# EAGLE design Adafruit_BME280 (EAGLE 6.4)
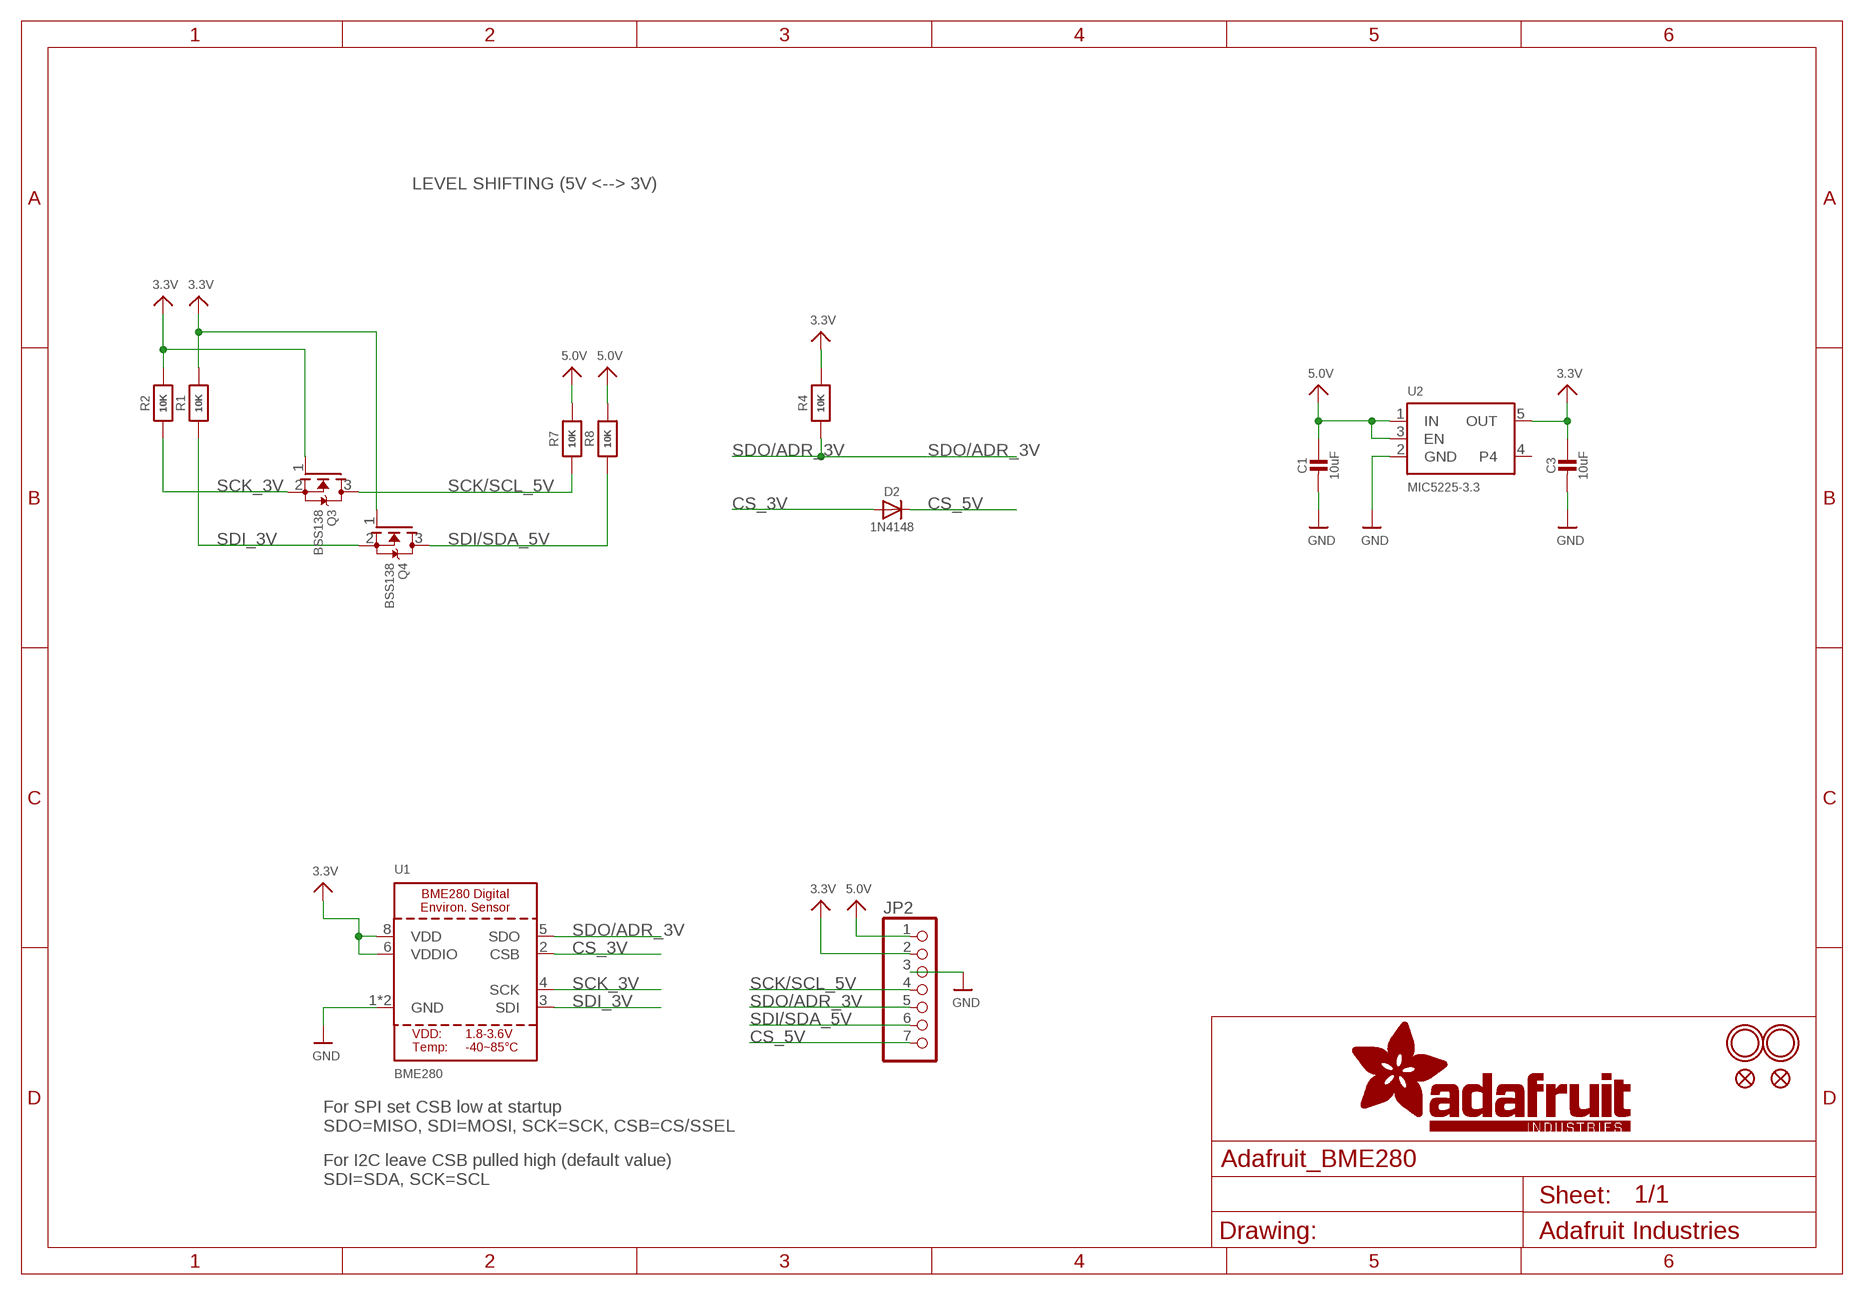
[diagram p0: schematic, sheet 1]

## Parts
C1  10uF  CAP_CERAMIC0805-NOOUTLINE  [0805-NO]
C3  10uF  CAP_CERAMIC0805-NOOUTLINE  [0805-NO]
D2  1N4148  DIODESOD-323  [SOD-323]
JP2  HEADER-1X770MIL  [1X07_ROUND_70]
Q3  BSS138  MOSFET-NWIDE  [SOT23-WIDE]
Q4  BSS138  MOSFET-NWIDE  [SOT23-WIDE]
R1  10K  RESISTOR0805_NOOUTLINE  [0805-NO]
R2  10K  RESISTOR0805_NOOUTLINE  [0805-NO]
R4  10K  RESISTOR_0805MP  [_0805MP]
R7  10K  RESISTOR0805_NOOUTLINE  [0805-NO]
R8  10K  RESISTOR0805_NOOUTLINE  [0805-NO]
U1  BME280  [BME280]
U2  MIC5225-3.3  VREG_SOT23-5  [SOT23-5]
U$5  FIDUCIAL""  [FIDUCIAL_1MM]
U$7  MOUNTINGHOLE2.0  [MOUNTINGHOLE_2.0_PLATED]
U$8  MOUNTINGHOLE2.0  [MOUNTINGHOLE_2.0_PLATED]
U$15  FIDUCIAL""  [FIDUCIAL_1MM]

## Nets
3.3V: C3.1 JP2.2 Q3.1(G) Q4.1(G) R1.2 R2.2 R4.2 U1.6(VDDIO) U1.8(VDD) U2.5(OUT)
5.0V: C1.1 JP2.1 R7.2 R8.2 U2.1(IN) U2.3(EN)
CS_3V: D2.A U1.2(CSB)
CS_5V: D2.C JP2.7
GND: C1.2 C3.2 JP2.3 U1.1(GND) U1.7(GND) U2.2(GND)
SCK/SCL_5V: JP2.4 Q3.3(D) R7.1
SCK_3V: Q3.2(S) R2.1 U1.4(SCK)
SDI/SDA_5V: JP2.6 Q4.3(D) R8.1
SDI_3V: Q4.2(S) R1.1 U1.3(SDI)
SDO/ADR_3V: JP2.5 R4.1 U1.5(SDO)
Unconnected: U2.4

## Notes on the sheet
- LEVEL SHIFTING (5V <--> 3V)
- For SPI set CSB low at startup
  SDO=MISO, SDI=MOSI, SCK=SCK, CSB=CS/SSEL
- For I2C leave CSB pulled high (default value)
  SDI=SDA, SCK=SCL

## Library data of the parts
C1 C3 = microbuilder:CAP_CERAMIC: Ceramic Capacitors
D2 = microbuilder:DIODE: Diode
JP2 = microbuilder:HEADER-1X7: PIN HEADER
Q3 Q4 = microbuilder:MOSFET-N: N-Channel Mosfet LEGEND VDS: Voltage Drain-Source ID: Drain Current RDS(ON): Drain-Source On-State Resistance VGS(TH): Gate-Source Threshold Voltage CISS: Drain-Source Input Capacitance SOT-23 Name VDS ID RDS(ON) VGS(TH) CISS Order Number 2N7002E 60V 260mA 2.5 Ohm 2.5V @ 250uA 26.7pF @ 25V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
R1 R2 R4 R7 R8 = microbuilder:RESISTOR: Resistors
U1 = microbuilder:BME280: BME280 - Environmental Sensor (I2C + SPI)
U2 = microbuilder:VREG_SOT23-5: SOT23-5 Fixed Voltage Regulators Part Current Out V Out V In V Dropout θJA (°C/W) TJ (°C) Digikey Part No. ADP121 150mA 3.3V 3.4-5.5V 0.09V @ 150mA -- -- ADP121-AUJZ33R7CT-ND ADP121 150mA 3.0V 3.1-5.5V 0.09V @ 150mA -- -- ADP121-AUJZ30R7CT-ND ADP122 300mA 3.3V 3.4-5.5V 0.085V @ 300mA -- --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
U$5 U$15 = microbuilder:FIDUCIAL: Fiducial Alignment Points; BOM: EXCLUDE
U$7 U$8 = microbuilder:MOUNTINGHOLE: Mounting Hole; BOM: EXCLUDE

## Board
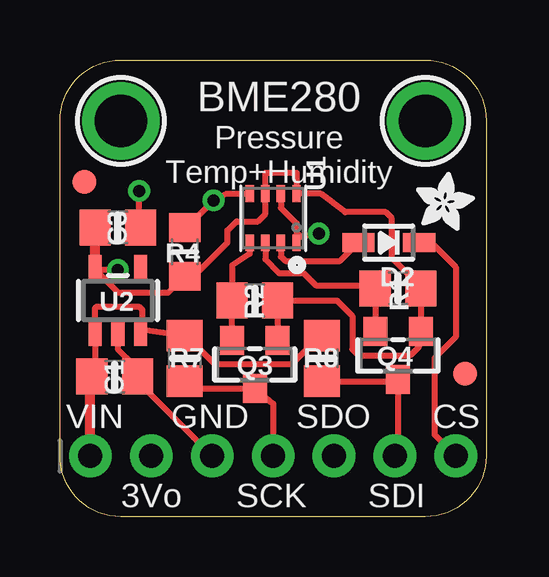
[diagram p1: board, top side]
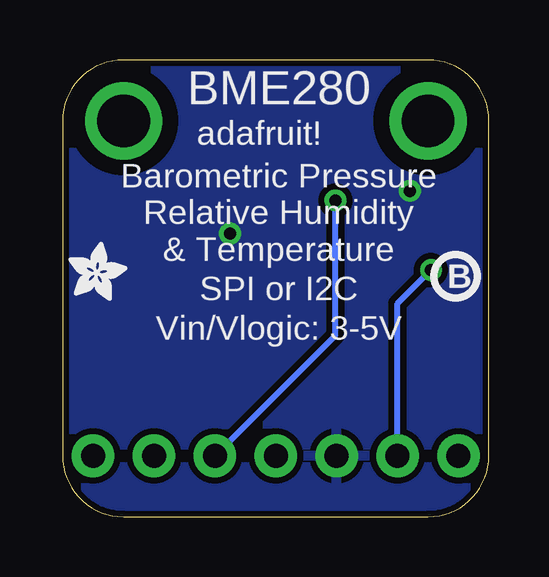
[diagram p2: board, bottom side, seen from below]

Size 17.78 x 19.05 mm. Coordinates in mm from the lower left corner, seen from the top.
Outline: 15.24,0 2.54,0 arc-90 0,2.54 0,16.51 arc-90 2.54,19.05 15.24,19.05 arc-90 17.78,16.51 17.78,2.54 arc-90 15.24,0
Copper layers (1*16): Top 0.035mm / dielectric 1.5mm / Bottom 0.035mm
Design rules "adafruit": minimum track width 8mil, minimum drill 15.5mil, track to track 8mil, track to pad 8mil, pad to pad 8mil, via to via 8mil, smd to smd 8mil, copper to edge 10mil, drill to drill 8mil, minimum pad ring 10mil, minimum via ring 8mil, stop-mask expansion 2mil, vias tented up to drill 20mil, thermal gap 10mil

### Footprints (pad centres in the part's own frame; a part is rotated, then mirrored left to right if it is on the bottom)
0805-NO = smd 1.3 x 1.5: 1 -0.95,0; 2 0.95,0
SOD-323 = smd 1.35 x 0.8: A 1.27,0; C -1.27,0
1X07_ROUND_70 = drill 1 pad 1.778: 1 -7.62,0; 2 -5.08,0; 3 -2.54,0; 4 0,0; 5 2.54,0; 6 5.08,0; 7 7.62,0
SOT23-WIDE = smd 1 x 1.2: 1 -0.95,-1; 2 0.95,-1; 3 0,1
_0805MP = smd 1.2 x 1.3: 1 -1.016,0; 2 1.016,0
BME280 = smd 0.7 x 0.35: 1 1.025,0.975; 2 1.025,0.325; 3 1.025,-0.325; 4 1.025,-0.975; 5 -1.025,-0.975; 6 -1.025,-0.325; 7 -1.025,0.325; 8 -1.025,0.975
SOT23-5 = smd 0.55 x 1.2: 1 -0.95,-1.3; 2 0,-1.3; 3 0.95,-1.3; 4 0.95,1.3; 5 -0.95,1.3
FIDUCIAL_1MM = smd 1 x 1: 1 0,0
MOUNTINGHOLE_2.0_PLATED = drill 2.2 pad 3: P$1 0,0

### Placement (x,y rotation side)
C1  2.29,5.84 0 top
C3  2.41,12.06 0 top
D2  13.72,11.43 180 top
JP2  8.89,2.54 0 top
Q3  8.13,6.35 180 top
Q4  14.1,6.73 180 top
R1  14.1,9.53 0 top
R2  8.13,9.02 0 top
R4  5.21,11.05 270 top
R7  5.21,6.6 90 top
R8  10.92,6.6 90 top
U1  8.89,12.45 270 top
U2  2.41,9.02 0 top
U$2  [ADAFRUIT_2.5MM]  17.53,9.02 0 bottom
U$5  1.02,13.97 0 top
U$6  [ADAFRUIT_2.5MM]  14.86,11.94 0 top
U$7  2.54,16.51 0 top
U$8  15.24,16.51 0 top
U$15  16.89,5.97 0 top
U$20  [PCBFEAT-REV-040]  1.4,10.03 0 bottom

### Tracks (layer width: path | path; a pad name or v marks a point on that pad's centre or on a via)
3.3V  (via drill 0.5)
  Top 0.254: Q3.1 R2.2 11.56,9.02 12.19,8.38 12.19,6.99 12.45,6.73 14.61,6.73 14.99,7.11 14.99,7.67 Q4.1 R1.2 15.05,9.59 13.84,10.79 13.84,12.45 13.59,12.7 11.91,12.7 10.88,13.47 U1.8 9.87,14.35 8.56,14.35 U1.6 8.56,12.63 8.26,12.32 7.37,12.32 6.99,11.94 6.99,11.43 5.59,10.03 R4.2 4.51,9.34 2.45,9.34 U2.5 1.49,10.29 v2.41,10.29
  Top 0.406: U2.5 C3.1
  Bottom 0.254: JP2.2 3.81,8.89 v2.41,10.29
5.0V
  Top 0.254: 3.43,7.78 3.43,8.64 3.3,8.76 1.52,8.76 1.46,8.7 U2.1 1.46,5.84 C1.1 1.27,5.84 1.27,5.65 | 3.43,7.78 U2.3 | 3.43,7.78 3.45,7.81 R7.2 5.27,7.55 6.48,6.35 9.65,6.35 10.98,7.68 R8.2
  Top 0.406: JP2.1 1.27,5.65
CS_3V
  Top 0.254: U1.2 9.21,10.85 9.4,10.67 11.68,10.67 D2.A
CS_5V
  Top 0.254: D2.C 15.49,11.43 16.51,10.41 16.51,7.49 15.62,6.6 15.62,3.43 JP2.7
GND  (via drill 0.5)
  Top 0.254: U1.7 9.21,12.88 9.87,12.23 9.87,11.86 | 9.87,11.86 U1.1 | C3.2 3.3,12.13 v3.3,13.59 | U2.2 2.41,6.99 3.05,6.35 3.05,6.03 C1.2 3.24,5.65 JP2.3 | 9.87,11.86 10.04,11.68 v10.79,11.81
  Bottom 0.254: v3.3,13.59 3.17,13.72 3.05,13.72 | v10.79,11.81 11.05,11.68
  pour Bottom (isolate 0.254): 0,19.05 17.78,19.05 17.91,0 0.13,0
SCK/SCL_5V
  Top 0.254: R7.1 5.64,5.35 Q3.3 8.89,4.71 JP2.4
SCK_3V
  Top 0.254: Q3.2 R2.1 7.18,10.48 7.92,10.96 U1.4
SDI/SDA_5V
  Top 0.254: JP2.6 14.1,2.67 Q4.3 14.05,5.65 R8.1
SDI_3V
  Top 0.254: Q4.2 R1.1 13.02,9.65 10.67,9.65 10.16,10.16 9.14,10.16 8.56,10.74 U1.3
SDO/ADR_3V  (via drill 0.5)
  Top 0.254: U1.5 6.93,13.47 v6.4,13.19 5.27,12.06 R4.1
  Bottom 0.254: JP2.5 6.4,7.57 v6.4,13.19

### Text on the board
tPlace: BME280 | Pressure / Temp+Humidity | VIN | GND | SDO | CS | 3Vo | SCK | SDI
bPlace: BME280 | adafruit! | Barometric Pressure / Relative Humidity / & Temperature | SPI or I2C | Vin/Vlogic: 3-5V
